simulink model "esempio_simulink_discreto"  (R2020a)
settings: Solver=VariableStepAuto  StartTime=0.0  StopTime=10000  RelTol=1e-3
undefined symbols (not defined in the file): den, num, Ts

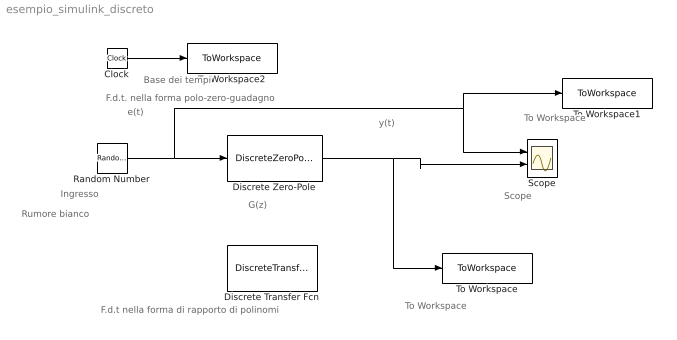
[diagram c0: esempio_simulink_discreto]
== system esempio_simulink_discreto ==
  note: F.d.t nella forma di rapporto di polinomi
  note: F.d.t. nella forma polo-zero-guadagno
  note: Base dei tempi
  note: To Workspace
  note: To Workspace
  note: Scope
  note: Rumore bianco
  note: G(z)
  note: y(t)
  note: Ingresso
  note: e(t)
  Clock : Clock
  Discrete Transfer Fcn : DiscreteTransferFcn  Numerator=num  Denominator=den  SampleTime=Ts
  Discrete Zero-Pole : DiscreteZeroPole  Zeros=[]  Poles=[0.2 0.5 0.3]  Gain=1  SampleTime=Ts
  Random Number : RandomNumber  SampleTime=Ts
  Scope : Scope  NumInputPorts=2
  To Workspace : ToWorkspace  VariableName=y  SampleTime=Ts
  To Workspace1 : ToWorkspace  VariableName=e  SampleTime=Ts
  To Workspace2 : ToWorkspace  VariableName=tsim  SampleTime=Ts
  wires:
  Random Number/1 -> To Workspace1/1, Scope/1, Discrete Zero-Pole/1
  Discrete Zero-Pole/1 -> To Workspace/1, Scope/2
  Clock/1 -> To Workspace2/1
